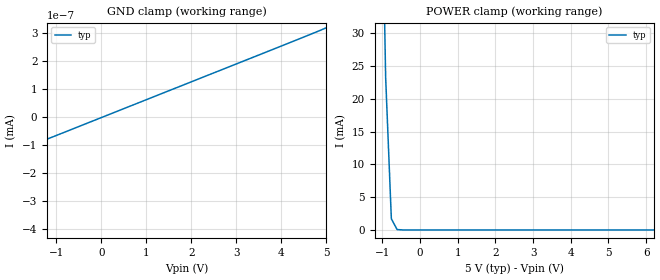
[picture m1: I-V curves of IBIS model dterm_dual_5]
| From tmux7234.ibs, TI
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| dterm_dual_5
[Model]   dterm_dual_5
Model_type   Terminator
|   typ   min   max
C_comp   1.008417e-11   NA   NA
[Voltage Range]   5   NA   NA
[Temperature Range]   27   NA   NA
[Power Clamp Reference]   5   NA   NA
[GND Clamp Reference]   0   NA   NA
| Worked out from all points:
|   GND clamp passes 1 mA (typ) near -5.69 V on its own axis
|   POWER clamp passes 1 mA (typ) near -0.69 V on its own axis
[GND Clamp]
|   Voltage   I(typ)   I(min)   I(max)
-10V      -2.315A    NA         NA
-5.152V   -619.7pA   NA         NA
-5V       -322pA     NA         NA
5V        318.9pA    NA         NA
[POWER Clamp]
|   Voltage   I(typ)   I(min)   I(max)
-5V       3.072A     NA         NA
-1.061V   70.97mA    NA         NA
-909.1mV  23.35mA    NA         NA
-757.6mV  1.704mA    NA         NA
-606.1mV  68.92uA    NA         NA
10V       -322pA     NA         NA
